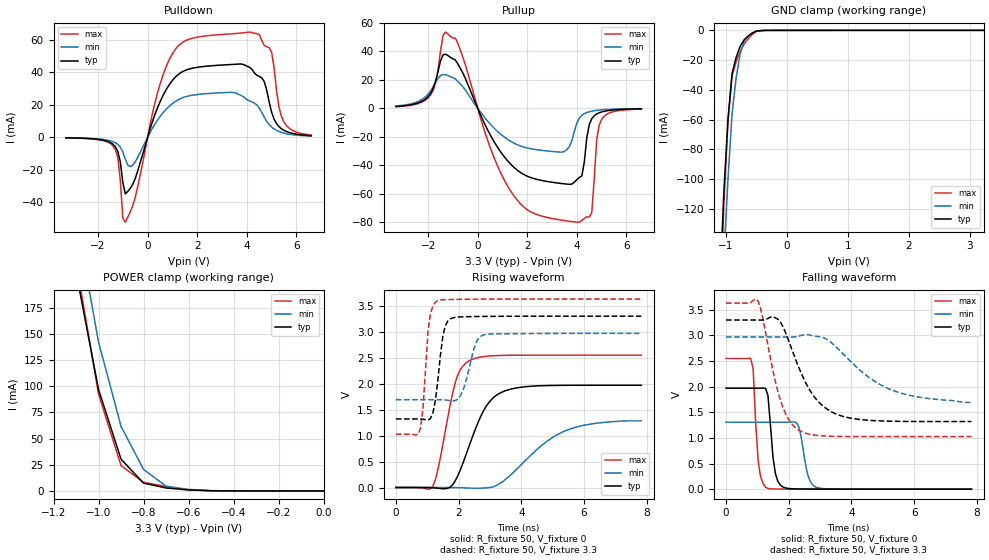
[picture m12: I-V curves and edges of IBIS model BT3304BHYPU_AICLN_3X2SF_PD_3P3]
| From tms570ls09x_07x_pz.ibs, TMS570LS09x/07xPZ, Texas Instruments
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|   Model Cell BT3304BHYPU_AICLN_3X2SF_PD_3P3
|BT3304BHYPU_AICLN_3X2SF_PD_3P3
[Model]   BT3304BHYPU_AICLN_3X2SF_PD_3P3
Model_type   I/O
Polarity   Non-Inverting
Enable   Active-Low
Vinl =  1.15
Vinh =  1.55
Cref =  15.0001pF
Rref =  101.0000M
Vref =  0V
Vmeas =  1.65
C_comp   1.2p   1.2p   1.2p
[Model Spec]
Vinl   1.15   1.02   1.28
Vinh   1.55   1.45   1.65
[Temperature Range]   25   155   -40
[Voltage Range]   3.3   2.97   3.63
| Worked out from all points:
|   slope of the pulldown table from 0 to 0.495 V, typ, clamps not added: 22.9 ohm
|   slope of the pullup table from 0 to 0.495 V, typ, clamps not added: 26.9 ohm
|   GND clamp passes 1 mA (typ) near -0.53 V on its own axis
|   POWER clamp passes 1 mA (typ) near -0.60 V on its own axis
|   rising waveform, R_fixture 50, V_fixture 0: 20-80 % time 801ps typ, 1.49ns min, 508ps max; typ from 0 V to 1.97 V
|   rising waveform, R_fixture 50, V_fixture 3.3: 20-80 % time 227ps typ, 333ps min, 180ps max; typ from 1.32 V to 3.3 V
|   falling waveform, R_fixture 50, V_fixture 0: 20-80 % time 181ps typ, 234ps min, 147ps max; typ from 1.97 V to 0 V
|   falling waveform, R_fixture 50, V_fixture 3.3: 20-80 % time 941ps typ, 1.62ns min, 605ps max; typ from 3.3 V to 1.32 V
[POWER_clamp]
|   voltage   I(typ)   I(min)   I(max)
-3.3V     3.99A      4.579A     4.788A
-1.1V     209.6mA    262.2mA    219.1mA
-1.067V   172.1mA    222.3mA    177mA
-1.033V   134.5mA    182.3mA    134.9mA
-1V       96.98mA    142.4mA    92.77mA
-900mV    30.41mA    61.81mA    24.23mA
-800mV    7.462mA    20.57mA    8.247mA
-700mV    2.848mA    4.595mA    4.228mA
-600mV    949.8uA    1.092mA    1.467mA
-500mV    155.7uA    238.9uA    226.8uA
0V        18.81uA    8.065uA    36.23uA
[Pulldown]
|   voltage   I(typ)   I(min)   I(max)
-3.3V     -317.2uA   -283uA     -323.2uA
-1.4V     -4.187mA   -2.645mA   -5.141mA
-1.2V     -8.732mA   -4.393mA   -12.51mA
-1V       -27.63mA   -8.973mA   -49.56mA
-900mV    -34.73mA   -13.26mA   -52.12mA
400mV     18.17mA    10.56mA    27.31mA
1.1V      36.68mA    21.82mA    53.65mA
4.1V      43.08mA    22.4mA     64.63mA
4.7V      34.41mA    12.54mA    56.53mA
5V        15.54mA    6.34mA     52.45mA
5.5V      4.314mA    2.594mA    9.388mA
6.6V      981uA      787.2uA    1.387mA
[Pullup]
|   voltage   I(typ)   I(min)   I(max)
-3.3V     1.246mA    1.609mA    1.076mA
-2V       8.232mA    9.997mA    7.367mA
-1.4V     37.5mA     23.8mA     51.32mA
-900mV    33.96mA    20.66mA    49.39mA
1.4V      -40.56mA   -23.96mA   -60.16mA
3.4V      -52.99mA   -30.87mA   -78.78mA
4V        -50.22mA   -10.35mA   -80.18mA
4.2V      -47.59mA   -4.955mA   -78.93mA
4.6V      -7.373mA   -1.996mA   -73.36mA
4.8V      -3.99mA    -1.436mA   -21.72mA
5V        -2.558mA   -1.08mA    -7.69mA
6.6V      -380.4uA   -267.9uA   -552uA
[GND_clamp]
|   voltage   I(typ)   I(min)   I(max)
-3.3V     -3.259A    -2.879A    -4.965A
-1.1V     -172mA     -209.5mA   -194.3mA
-1.033V   -107.5mA   -151.2mA   -115.6mA
-966.7mV  -59.82mA   -100mA     -61.12mA
-900mV    -29.02mA   -56.02mA   -30.69mA
-833.3mV  -18.2mA    -32.15mA   -21.26mA
-766.7mV  -10.63mA   -15.71mA   -14.05mA
-700mV    -6.316mA   -6.699mA   -9.091mA
-566.7mV  -1.768mA   -1.723mA   -2.661mA
-500mV    -462.1uA   -565.3uA   -689.4uA
-366.7mV  -25.67uA   -48.26uA   -36.28uA
3.233V    18.8uA     10.51uA    36.2uA
[Ramp]
| variable   typ   min   max
dV/dt_f   1.227724/0.9519912n   0.792894/1.639654n   1.6126/0.6128399n
dV/dt_r   1.196428/0.8084009n  0.7931546/1.548924n   1.548914/0.5103091n
R_load = 50
[Rising Waveform]
R_fixture = 50
V_fixture = 0
V_fixture_min = 0
V_fixture_max = 0
|   time   V(typ)   V(min)   V(max)
0s        -1.491uV   -134.8nV   -3.57uV
1.18ns    -5.676mV   -5.538uV   28.35mV
1.336ns   -13.29mV   17.17uV    338.5mV
1.888ns   125mV      -992.9uV   2.011V
2.04ns    319mV      -3.384mV   2.253V
2.34ns    808.3mV    -10.46mV   2.441V
2.896ns   1.581V     -7.179mV   2.529V
3.464ns   1.859V     139.9mV    2.545V
5.396ns   1.968V     1.091V     2.549V
7.828ns   1.97V      1.283V     2.549V
[Rising Waveform]
R_fixture = 50
V_fixture = 3.3
V_fixture_min = 2.97
V_fixture_max = 3.63
|   time   V(typ)   V(min)   V(max)
0s        1.32V      1.692V     1.025V
784ps     1.319V     1.692V     1.142V
864ps     1.315V     1.692V     1.533V
1.024ns   1.298V     1.692V     3.011V
1.18ns    1.439V     1.692V     3.501V
1.336ns   2.055V     1.692V     3.598V
1.572ns   3.107V     1.686V     3.618V
1.808ns   3.266V     1.667V     3.622V
2.796ns   3.295V     2.938V     3.629V
7.828ns   3.3V       2.97V      3.63V
[Falling Waveform]
R_fixture = 50
V_fixture = 0
V_fixture_min = 0
V_fixture_max = 0
|   time   V(typ)   V(min)   V(max)
0s        1.97V      1.306V     2.549V
784ps     1.97V      1.306V     2.551V
864ps     1.97V      1.306V     2.353V
1.024ns   1.969V     1.306V     551.9mV
1.336ns   1.828V     1.306V     12.72mV
1.572ns   311mV      1.306V     3.82mV
1.808ns   44.22mV    1.306V     2.51mV
2.292ns   4.708mV    1.255V     968.8uV
2.896ns   1.995mV    32.96mV    224uV
7.828ns   15.7uV     228.7uV    18.31uV
[Falling Waveform]
R_fixture = 50
V_fixture = 3.3
V_fixture_min = 2.97
V_fixture_max = 3.63
|   time   V(typ)   V(min)   V(max)
0s        3.3V       2.97V      3.63V
1.024ns   3.3V       2.97V      3.667V
1.732ns   3.262V     2.97V      1.739V
2.04ns    2.825V     2.969V     1.319V
2.34ns    2.346V     2.99V      1.143V
2.896ns   1.739V     2.98V      1.05V
3.692ns   1.426V     2.664V     1.028V
4.604ns   1.342V     2.158V     1.026V
5.396ns   1.324V     1.908V     1.026V
7.828ns   1.32V      1.692V     1.025V
